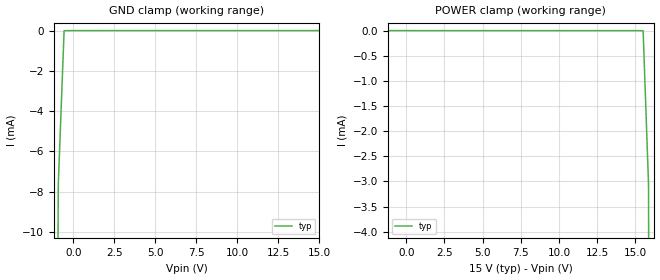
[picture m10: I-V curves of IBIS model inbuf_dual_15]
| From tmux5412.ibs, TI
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| inbuf_dual_15
[Model]   inbuf_dual_15
Model_type   Input
Vinl = 0.8
Vinh = 1.3
|   typ   min   max
C_comp   2.533030e-12   NA   NA
[Voltage Range]   15   NA   NA
[Temperature Range]   27   NA   NA
[Power Clamp Reference]   15   NA   NA
[GND Clamp Reference]   0   NA   NA
[GND Clamp]
|   Voltage   I(typ)   I(min)   I(max)
-20V      -18.62A    NA         NA
-1.263V   -62.84mA   NA         NA
-909.1mV  -7.638mA   NA         NA
-555.6mV  -6.629uA   NA         NA
15V       683.9nA    NA         NA
[POWER Clamp]
|   Voltage   I(typ)   I(min)   I(max)
-5V       1.224uA    NA         NA
15.51V    -2.633uA   NA         NA
15.86V    -3.059mA   NA         NA
16.21V    -54.11mA   NA         NA
30V       -11.55A    NA         NA
